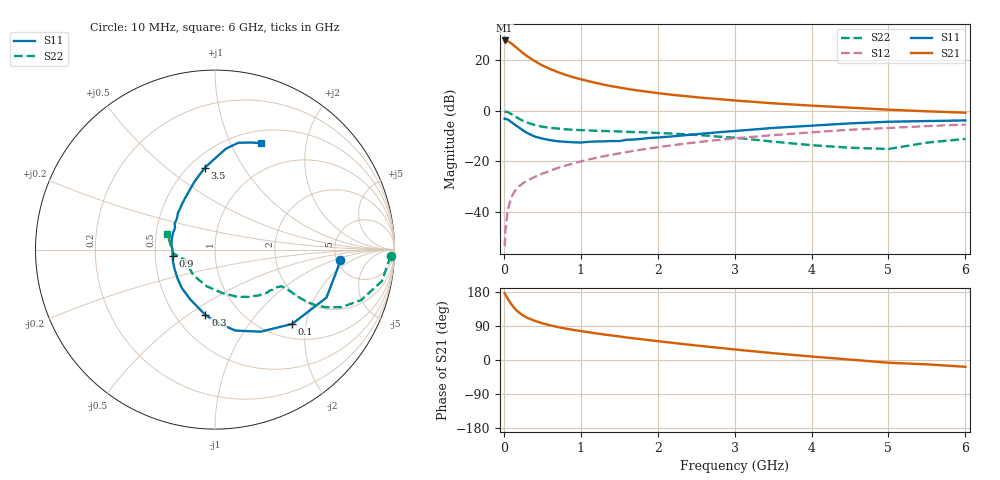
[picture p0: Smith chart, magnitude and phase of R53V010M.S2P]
! SIEMENS Small Signal Semiconductors
! BFR183
! Si NPN RF Bipolar Junction Transistor in SOT23
! VCE = 3 V  IC = 10 mA
! Common Emitter S-Parameters:  May  1996
# GHz  S  MA  R  50
!  f  S11  S21  S12  S22
! GHz  MAG  ANG  MAG  ANG  MAG  ANG  MAG  ANG
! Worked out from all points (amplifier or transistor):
!   36 points, 10 MHz to 6 GHz, reference 50 ohm
!   highest |S21| = 27.9 dB at 10 MHz (marker M1)
!   |S21| within 3 dB of that: start of sweep to 170.8 MHz
!   unconditionally stable (mu >= 1): 768.2 MHz to 2.507 GHz
!   at 250 MHz: K = 0.62, MSG = 25.7 dB, |S12| = -28.6 dB
!   at 1.4 GHz: K = 1.06, MAG = 12.1 dB, |S12| = -17.4 dB
!   at 6 GHz: K = 0.89, MSG = 2.4 dB, |S12| = -5.4 dB
!   lowest NFmin = 1.30 dB at 450 MHz
!   S11 on the Smith chart (normalised r, x): 10 MHz: 5.35, -1.25; 100 MHz: 1.30, -1.67; 300 MHz: 0.70, -0.59; 900 MHz: 0.62, -0.04; 3.5 GHz: 0.60, +0.69; 6 GHz: 0.64, +1.32
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0.01  0.6996 -4.9  24.77 176.3  0.0021 87.7  0.9797 -2.1
0.02  0.6896 -9.4  24.52 172.4  0.0042 86.5  0.9686 -4.3
0.05  0.6762 -23.3  24.05 162.0  0.0109 78.9  0.9461 -10.7
0.1  0.5971 -43.9  21.54 146.6  0.0199 71.0  0.8611 -19.1
0.15  0.5231 -61.0  18.61 133.8  0.0271 66.3  0.7737 -24.5
0.2  0.4654 -75.8  16.12 124.6  0.0322 64.1  0.6952 -27.5
0.25  0.4101 -87.7  13.89 117.4  0.0371 62.3  0.6341 -29.0
0.3  0.3679 -98.4  12.17 111.7  0.0414 62.4  0.5901 -29.6
0.4  0.3111 -115.8  9.703 103.5  0.0491 62.9  0.5258 -29.6
0.5  0.2832 -130.7  7.94 96.8  0.0571 63.9  0.4856 -29.1
0.6  0.2635 -142.4  6.754 91.7  0.0653 64.5  0.4622 -28.8
0.7  0.2505 -153.6  5.875 87.1  0.0741 65.2  0.4469 -28.7
0.9  0.2388 -172.0  4.648 79.6  0.0913 65.7  0.4229 -28.9
1.1  0.2438 174.4  3.875 73.4  0.1085 65.4  0.4097 -30.6
1.3  0.2493 161.9  3.306 67.5  0.1267 64.6  0.3999 -32.2
1.6  0.2683 147.0  2.731 59.3  0.1536 62.9  0.3848 -36.0
2.2  0.3141 125.6  2.069 45.1  0.2099 58.1  0.3557 -45.7
2.8  0.3787 109.6  1.706 32.1  0.2674 51.9  0.3086 -58.4
3.5  0.4597 97.1  1.412 18.0  0.3311 43.3  0.2463 -80.1
4.5  0.5656 83.8  1.16 1.1  0.4234 31.0  0.1865 -130.9
5.5  0.6292 71.4  0.98 -11.5  0.5003 19.0  0.2354 -175.1
6  0.6475 66.5  0.921 -18.0  0.536 11.3  0.2785 161.9
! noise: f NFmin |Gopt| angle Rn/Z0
0.45  1.3  0.15  45  0.18
0.9  1.4  0.2  125  0.19
1.8  2.1  0.34  -170  0.14
